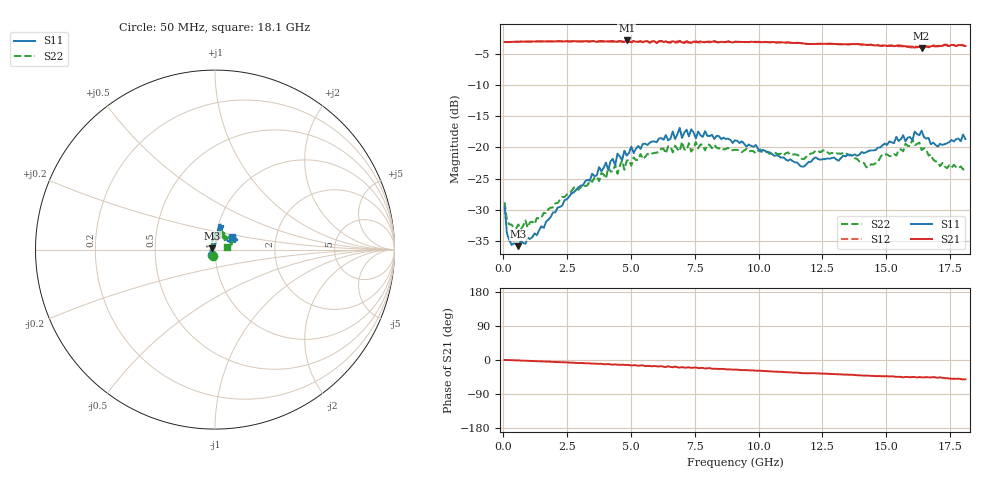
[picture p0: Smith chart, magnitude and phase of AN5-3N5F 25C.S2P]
! Network Analyzer HP8720D.06.14 Serial No. US36140669
! 27 Jun 2005  11:05:40
! Frequency  S11  S21  S12  S22
# HZ  S  DB R 50
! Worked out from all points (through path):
!   201 points, 50 MHz to 18.1 GHz, reference 50 ohm
!   highest |S21| = -2.91 dB at 4.833 GHz (marker M1); lowest = -4.1 dB at 16.39 GHz (marker M2)
!   group delay of S21, straight-line fit = 7.97 ps
!   lowest |S11| = -35.8 dB at 591.5 MHz (marker M3), VSWR 1.03, Z = 48.6 + j0.808 ohm
!   |S11| at or under -10 dB: start of sweep to end of sweep
!   |S22| runs from -33.1 to -18.7 dB; largest |S21 - S12| = 0.025
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5e7  -29.41 -120.2  -3.15 0.0  -3.15 0.2  -28.78 -108.0
1.4025e8  -33.73 -152.3  -3.17 -0.1  -3.16 -0.0  -31.59 -156.2
5.915e8  -35.79 149.2  -3.10 -1.1  -3.11 -1.1  -32.33 161.2
1.22325e9  -33.74 118.2  -3.07 -2.9  -3.08 -2.9  -32.25 135.7
3.1185e9  -26.05 79.9  -3.06 -8.1  -3.08 -8.3  -25.95 107.3
4.83325e9  -21.31 78.0  -2.91 -13.0  -3.03 -13.6  -22.13 85.2
6.09675e9  -18.57 73.3  -3.07 -17.1  -3.00 -16.8  -20.71 79.0
6.7285e9  -18.68 79.0  -3.14 -17.4  -3.30 -18.2  -19.73 71.1
6.909e9  -16.87 77.5  -2.96 -20.1  -3.06 -18.9  -20.62 69.6
6.99925e9  -18.50 76.5  -3.20 -19.1  -3.28 -20.4  -19.11 70.9
7.36025e9  -17.09 70.4  -3.32 -20.8  -3.13 -20.0  -20.68 74.3
7.54075e9  -18.55 72.2  -3.15 -19.6  -3.03 -21.5  -19.14 73.2
9.075e9  -18.87 79.5  -3.13 -25.3  -3.10 -25.4  -20.37 56.4
1.169225e10  -23.10 65.6  -3.36 -34.6  -3.35 -34.5  -21.84 52.1
1.21435e10  -21.82 62.6  -3.47 -34.7  -3.43 -34.9  -20.89 56.2
1.3407e10  -21.45 44.8  -3.52 -38.4  -3.50 -38.5  -20.82 49.7
1.421925e10  -20.76 27.9  -3.61 -40.9  -3.60 -41.1  -23.18 47.9
1.512175e10  -19.06 23.7  -3.79 -43.5  -3.67 -43.3  -21.39 47.4
1.602425e10  -18.86 28.2  -3.87 -44.7  -4.06 -46.4  -18.71 32.7
1.638525e10  -17.32 23.5  -4.11 -45.5  -3.87 -45.1  -20.43 21.6
1.7017e10  -19.88 28.9  -3.75 -47.0  -3.89 -48.0  -22.36 15.9
1.81e10  -18.66 37.3  -3.79 -50.8  -3.84 -51.4  -23.31 11.7
